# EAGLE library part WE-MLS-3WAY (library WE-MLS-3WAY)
Multiline EMI Suppression Ferrite - Filter for common mode or differential mode - High rated current with typ. 4 A - High impedance common mode inductor with 2x2 winding made by PCB line connection - Broardband litering because of the NiZn-ferrite core - RF- common mode inductor for 2,3 or 4 lines in one component -- Perfect suitable for absorption of common or differential mode interferences in the field of EMC -- High current DC output filters of power supplies e.g. battery chargers, industrial power supplies -- With one turn the component performes like a 3 or 4 times common mode chock for the signal
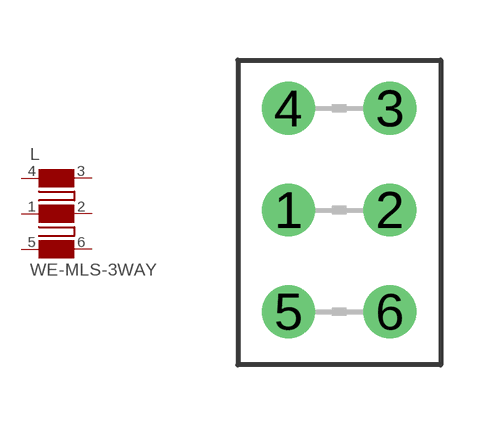
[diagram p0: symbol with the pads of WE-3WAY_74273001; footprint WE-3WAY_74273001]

Designator prefix L

## WE-MLS-3WAY_74273001, WE-MLS-3WAY-74273001_74273001 (MPN: 74273001; OC_FARNELL: 1635786; OC_NEWARK: 08P2348; PACKAGE: 74273002x; SUPPLIER: Wuerth Elektronik)  [WE-3WAY_74273001]
1  2  pas
2  5  pas
3  6  pas
4  1  pas
5  3  pas
6  4  pas

## Footprint WE-3WAY_74273001 (pad centres in mm)
Multiline EMI Suppression Ferrite WE-MLS
drill 0.813: 1 -1.27,0; 2 1.27,0; 3 1.27,2.54; 4 -1.27,2.54; 5 -1.27,-2.54; 6 1.27,-2.54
